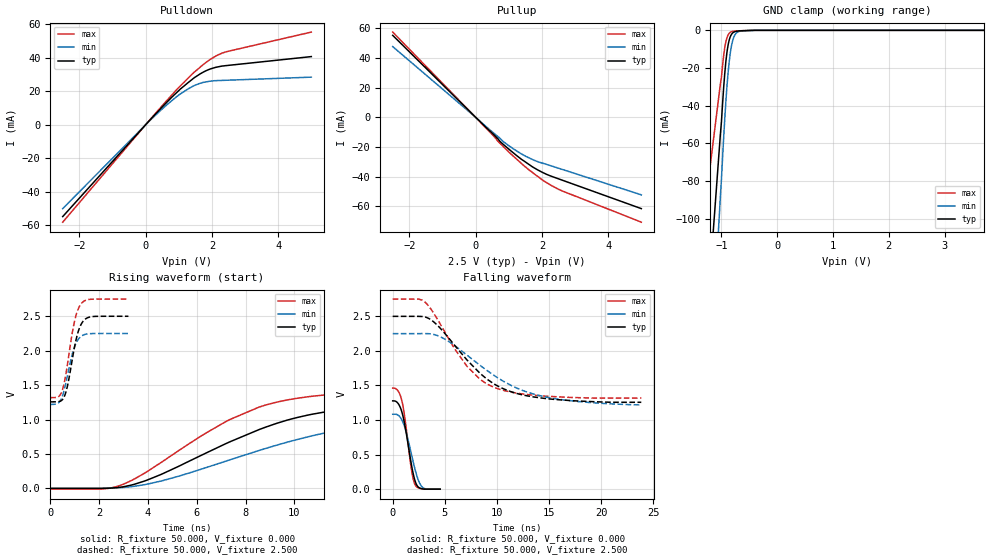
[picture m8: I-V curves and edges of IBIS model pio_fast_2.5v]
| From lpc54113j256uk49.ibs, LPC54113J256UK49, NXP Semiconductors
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[Model]   pio_fast_2.5v
Model_type I/O
Vinl=4.000E-01
Vinh=1.500E+00
Vref=0.000E+00
Rref=1.000E+06
Cref=2.000E-11
Vmeas=1.250E+00
C_comp   9.060E-12   8.700E-12   9.420E-12
[Voltage Range]   2.500E+00   2.250E+00   2.750E+00
[POWER Clamp Reference]   2.500E+00   2.250E+00   2.750E+00
[GND Clamp Reference]   0.000E+00   0.000E+00   0.000E+00
[Pullup Reference]   2.500E+00   2.250E+00   2.750E+00
[Pulldown Reference]   0.000E+00   0.000E+00   0.000E+00
[Temperature Range]   25   105   -40
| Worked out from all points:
|   slope of the pulldown table from 0 to 0.375 V, typ, clamps not added: 46.9 ohm
|   slope of the pullup table from 0 to 0.375 V, typ, clamps not added: 46.2 ohm
|   GND clamp passes 1 mA (typ) near -0.78 V on its own axis
|   rising waveform, R_fixture 50.000, V_fixture 0.000: 20-80 % time 5.17ns typ, 6.52ns min, 4.28ns max; typ from 0 V to 1.28 V
|   falling waveform, R_fixture 50.000, V_fixture 0.000: 20-80 % time 885ps typ, 1.06ns min, 766ps max; typ from 1.28 V to 0 V
|   rising waveform, R_fixture 50.000, V_fixture 2.500: 20-80 % time 409ps typ, 413ps min, 406ps max; typ from 1.26 V to 2.5 V
|   falling waveform, R_fixture 50.000, V_fixture 2.500: 20-80 % time 4.91ns typ, 6.27ns min, 4.01ns max; typ from 2.5 V to 1.26 V
[GND Clamp]
-2.5V     -652.6mA   -859.5mA   -381.3mA
-1.02V    -55.58mA   -88.8mA    -28.68mA
-1V       -48.54mA   -79.04mA   -24.92mA
-960mV    -30.29mA   -56.85mA   -13.33mA
-920mV    -16.37mA   -37.46mA   -5.921mA
-880mV    -7.654mA   -22.27mA   -2.388mA
-860mV    -5.02mA    -16.43mA   -1.529mA
-820mV    -2.133mA   -8.185mA   -717.9uA
-780mV    -993.5uA   -3.731mA   -464.6uA
-740mV    -551.3uA   -1.652mA   -372.6uA
-540mV    -121.9uA   -152.7uA   -101.6uA
5V        0A         0A         0A
[Power Clamp]
-2.5V     0A         0A         0A
0V        0A         0A         0A
2.5V      0A         0A         0A
5V        0A         0A         0A
[Pullup]
-2.5V     55.17mA    47.6mA     57.37mA
0V        0A         0A         0A
820mV     -17.99mA   -16.12mA   -19.39mA
1.4V      -28.61mA   -24.91mA   -31.48mA
1.94V     -36.26mA   -30.42mA   -40.98mA
2.26V     -39.55mA   -32.62mA   -45.65mA
2.54V     -41.8mA    -34.63mA   -48.95mA
5V        -61.57mA   -52.31mA   -70.72mA
[Pulldown]
-2.5V     -54.85mA   -50.1mA    -58.2mA
0V        0A         0A         0A
500mV     10.6mA     9.452mA    11.41mA
1.04V     21.22mA    18.33mA    23.13mA
1.42V     27.38mA    22.99mA    30.62mA
1.64V     30.38mA    24.79mA    34.37mA
1.84V     32.48mA    25.72mA    37.54mA
2.12V     34.38mA    26.41mA    41.13mA
2.44V     35.42mA    26.64mA    43.72mA
5V        40.78mA    28.5mA     55.43mA
[Rising Waveform]
R_fixture = 50.000
V_fixture = 0.000
V_fixture_min = 0.000
V_fixture_max = 0.000
|  time   V(typ)   V(min)   V(max)
0s        0V         0V         -10.9mV
2.1ns     -27.45uV   1.132mV    -9.946mV
2.9ns     18.24mV    11.18mV    47.42mV
4.5ns     196.8mV    103.6mV    367mV
7.35ns    675.7mV    414.1mV    999.4mV
8.6ns     860.5mV    555.9mV    1.186V
9.85ns    1.006V     685mV      1.294V
11.6ns    1.129V     831.4mV    1.368V
14.65ns   1.22V      976.5mV    1.423V
23.65ns   1.277V     1.084V     1.452V
[Falling Waveform]
R_fixture = 50.000
V_fixture = 0.000
V_fixture_min = 0.000
V_fixture_max = 0.000
|  time   V(typ)   V(min)   V(max)
0s        1.277V     1.084V     1.461V
500ps     1.243V     1.073V     1.424V
900ps     1.106V     994.4mV    1.264V
1.2ns     896.9mV    873.5mV    991.3mV
1.8ns     351.7mV    502.4mV    281.1mV
1.95ns    234.8mV    404.8mV    158.6mV
2.15ns    117.3mV    282.3mV    64.37mV
2.55ns    19.85mV    97.38mV    13.36mV
2.9ns     3.814mV    22.21mV    2.996mV
4.55ns    0V         0V         0V
[Rising Waveform]
R_fixture = 50.000
V_fixture = 2.500
V_fixture_min = 2.250
V_fixture_max = 2.750
|  time   V(typ)   V(min)   V(max)
0s        1.257V     1.22V      1.318V
400ps     1.265V     1.268V     1.355V
500ps     1.289V     1.344V     1.432V
600ps     1.355V     1.47V      1.581V
750ps     1.566V     1.718V     1.912V
950ps     1.972V     2.011V     2.354V
1.1ns     2.223V     2.14V      2.565V
1.25ns    2.374V     2.205V     2.675V
1.65ns    2.492V     2.248V     2.747V
3.2ns     2.5V       2.25V      2.75V
[Falling Waveform]
R_fixture = 50.000
V_fixture = 2.500
V_fixture_min = 2.250
V_fixture_max = 2.750
|  time   V(typ)   V(min)   V(max)
0s        2.5V       2.25V      2.75V
2.5ns     2.5V       2.25V      2.749V
3.1ns     2.491V     2.251V     2.705V
4.7ns     2.305V     2.195V     2.352V
7.1ns     1.873V     1.942V     1.783V
8.35ns    1.68V      1.795V     1.593V
9.7ns     1.524V     1.648V     1.475V
12.25ns   1.371V     1.44V      1.381V
14.9ns    1.307V     1.327V     1.343V
23.85ns   1.257V     1.22V      1.318V
[Ramp]
dV/dt_r   7.6469E-01/5.1563E-09   6.4858E-01/6.5173E-09   8.7806E-01/4.2483E-09
dV/dt_f   7.4600E-01/4.9050E-09   6.1833E-01/6.2646E-09   8.5930E-01/3.9848E-09
R_load = 50
